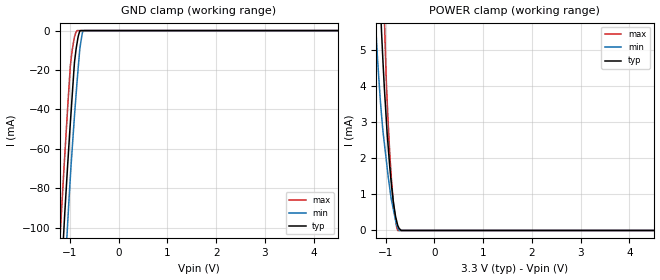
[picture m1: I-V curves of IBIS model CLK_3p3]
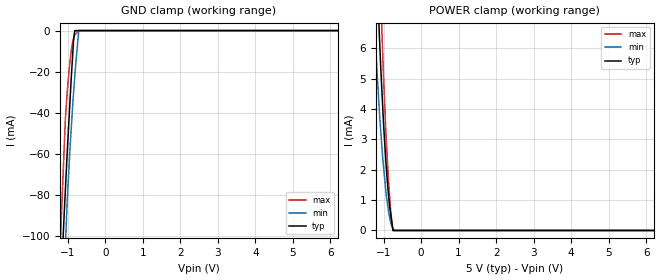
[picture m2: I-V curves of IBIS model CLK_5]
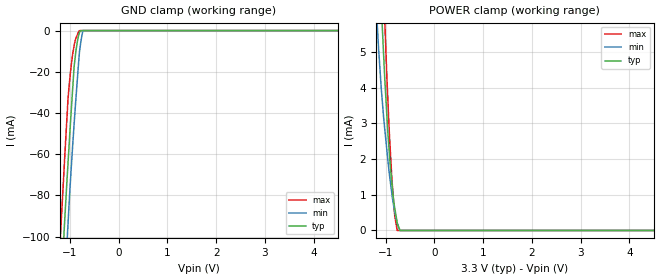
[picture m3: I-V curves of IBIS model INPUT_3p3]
|Texas Instruments Incorporated
|20 Bit Delta Sigma ADC for Bridge Sensors
| Marketing part#   Digital Voltage Range   Package-type   #pins
| ADS1230IPW   2.7V to 5.3V   TSSOP   16
| ADS1230IPWG4   2.7V to 5.3V   TSSOP   16
| ADS1230IPWR   2.7V to 5.3V   TSSOP   16
| ADS1230IPWRG4   2.7V to 5.3V   TSSOP   16
[IBIS Ver]   3.2
[File name]   ads1230.ibs
[Date]   07/16/2010
[File Rev]   1.2
[Source]
| Texas Instruments Incorporated.
| Analog eLab Design Center, HPA
| 12500 TI Blvd
| Dallas, TX -75243
| e-Mail: elab_scm_ibis@list.ti.com
| Model generated from simulations in TISPICE
[Notes]   Revision_History:
|   Rev 1.0: 05/25/2010
|   - Initial version of the model
|   - Initial Model generated from simulations in TIspiceD
|   - Model names with a trailing _3p3 contains the model for
|   3.3V [3 - 3.3 - 3.6]. Model names with trailing _5 contains
|   the model for 5V [4.75 - 5.0 - 5.25] operation.
|   Rev 1.1: 07/08/2010
|   - Model generated from simulations in TISPICE
|   - Model matched to SPICE simulation
|   - Updated the ibis file with data sheet title and package
|   details
|   - While calculating R_pkg, L_pkg and C_pkg ignored values
|   corresponding to power and ground pins
|   - Added package details beside [Package]
|   - C_comp although listed in numerical order of value are
|   obtained from varying PVT conditions. For PVT conditions
|   for each specific value refer the buffer description under
|   respective [Model]. IBIS model user is responsible for using
|   appropriate C_comp to simulate for Signal Integrity.
|   - Removed C_comp (ON state) and C_comp (OFF state) lines
|   Rev 1.2: 07/16/2010
|   - Updated the ibis file with Vinl and Vinh values calculated
|   using VDD typ values and also added model spec
|   - Added C_comp (ON state) and C_comp (OFF state) for OUTPUT_3p3
|   and OUTPUT_5 models
|   - Removed the out of range(-VDD to 2*VDD) voltages for clamp
|   and IV curves
[Disclaimer]
| This model is designed as an aid for customers of Texas Instruments.
| TI and its licensors and suppliers make no warranties, either expressed
| or implied, with respect to this  model, including the warranties of
| merchantability or fitness for a particular purpose. The model is
| provided solely on an "as is" basis. The entire risk as to its quality
| and performance is with the customer.
[Copyright]
| (C) Copyright 2010 Texas Instruments Incorporated. All rights reserved.
|   ADS1230
[Component]   ADS1230
[Manufacturer]  TI
[Package]  | 16 TSSOP - PW package
| variable   typ   min   max
R_pkg   0.07499   0.06418   0.0858
L_pkg   2.774805nH   2.2398nH   3.30981nH
C_pkg   0.48029pF   0.44652pF   0.51406pF
|-------------------------PIN------------------------------------------------
[Pin]  signal_name model_name   R_pin   L_pin   C_pin
1   DVDD   POWER   0.07591   3.10169nH   0.50422pF
2   DGND   GND   0.08317   2.62701nH   0.45709pF
3   CLKIN   CLK   0.06418   2.24125nH   0.45226pF
4   GAIN   INPUT   0.06418   2.23980nH   0.45110pF
5   CAP   TERM   0.06537   2.26241nH   0.45379pF
6   CAP   TERM   0.06501   2.25855nH   0.45528pF
7   AINP   TERM   0.07204   2.40738nH   0.44652pF
8   AINN   TERM   0.06723   2.93633nH   0.49461pF
9   REFN   TERM   0.08580   3.30981nH   0.51406pF
10   REFP   TERM   0.08477   2.66411nH   0.46463pF
11   AGND   GND   0.03843   2.07247nH   0.50509pF
12   AVDD   POWER   0.06944   2.34570nH   0.45854pF
13   SPEED   INPUT   0.06997   2.35644nH   0.46010pF
14   _PDWN   INPUT   0.06418   2.24133nH   0.45470pF
15   SCLK   INPUT   0.08390   2.64189nH   0.45754pF
16   _DRDY/DOUT  OUTPUT   0.07852   3.15400nH   0.50637pF
|   Model Selectors
[Model Selector]  CLK
CLK_3p3   3V digital input
CLK_5   5V digital input
|NOTES   Model CLK split into two Models CLK_3p3 and CLK_5
|   to accomodate vast voltage range of 2.7V - 5.3V
|   CLK_3p3 operates in voltage range of 3.0 - 3.3 - 3.6
|   CLK_5 operates in voltage range of 4.75 - 5.0 - 5.25
|   The max pin frequency for Model CLK is 6MHz
|   This is referenced with CLKIN pin in datasheet
[Model Selector]  INPUT
INPUT_3p3  3V digital input
INPUT_5   5V digital input
|NOTES   Model INPUT split into two Models INPUT_3p3 and INPUT_5
|   to accomodate vast voltage range of 2.7V - 5.3V
|   INPUT_3p3 operates in voltage range of 3.0 - 3.3 - 3.6
|   INPUT_5 operates in voltage range of 4.75 - 5.0 - 5.25
|   The max pin frequency for Model INPUT is 5MHz
|   This is referenced with SCLK pin in datasheet
[Model Selector]  OUTPUT
OUTPUT_3p3   3V digital output
OUTPUT_5   5V digital output
|NOTES   Model OUTPUT split into two Models OUTPUT_3p3 and OUTPUT_5
|   to accomodate vast voltage range of 2.7V - 5.3V
|   OUTPUT_3p3 operates in voltage range of 3.0 - 3.3 - 3.6
|   OUTPUT_5 operates in voltage range of 4.75 - 5.0 - 5.25
|   The max pin frequency for Model OUTPUT is 2.5MHz
|   This is referenced with timing diagrams of _DRDY/DOUT pin
|   in datasheet
|   TERM Model
[Model] TERM
Model_type Terminator
C_comp   0   0   0
| variable   typ   min   max
[Voltage Range]   3.3V   2.7V   5.3V
[POWER Clamp Reference]  3.3V   2.7V   5.3V
[GND Clamp Reference]   0.0V   0.0V   0.0V
|Operating Temperature
[Temperature Range]   25   85   -40
| Models and submodels in the file (7): TERM (Terminator), CLK_3p3 (Input), CLK_5 (Input), INPUT_3p3 (Input), INPUT_5 (Input), OUTPUT_3p3 (Output), OUTPUT_5 (Output)
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|   CLK INPUT 3V Model
[Model]   CLK_3p3
Model_type Input
| Signals  CLK
Vinl = 0.66
Vinh = 2.31
|   typ   min   max
|   (nom PVT)   (Fast PVT)   (slow PVT)
|Average
C_comp   1.099e-12   1.076e-12   1.134e-12
| Where   nom PVT is  Nominal Process, 3.3V, 25C
|   Fast PVT is Strong Process, 3.6V, -40C
|   Slow PVT is Weak Process, 3.0V, 85C
[model spec]
Vinl   0.66   0.6   0.72
Vinh   2.31   2.1   2.52
[Voltage Range]   3.3   3   3.6
|Ambient Temperature   25   85   -40
|Junction Temperature
[Temperature Range]   25   85   -40
[Power Clamp Reference]   3.3   3   3.6
[GND Clamp Reference]   0   0   0
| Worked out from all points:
|   GND clamp passes 1 mA (typ) near -0.81 V on its own axis
|   POWER clamp passes 1 mA (typ) near -0.86 V on its own axis
[GND Clamp]
|   Voltage   I(typ)   I(min)   I(max)
-3.3V     -1.171A    -1.197A    -1.147A
-1.191V   -132.1mA   -162.7mA   -99.85mA
-1.118V   -98.63mA   -129.9mA   -68.62mA
-1.056V   -72.27mA   -102.2mA   -43.23mA
-992.4mV  -47.42mA   -74.93mA   -18.44mA
-978mV    -42.17mA   -69.13mA   -15.05mA
-907.5mV  -16.46mA   -43.73mA   -3.436mA
-848.4mV  -5.674mA   -24.53mA   0A
-795mV    -229.2uA   -8.925mA   0A
-744mV    0A         -1.21mA    0A
-709.5mV  0A         0A         0A
6.6V      0A         0A         0A
[POWER Clamp]
|   Voltage   I(typ)   I(min)   I(max)
-3.3V     108.4mA    89.11mA    133.8mA
-1.201V   9.77mA     5.568mA    14.15mA
-1.164V   8.324mA    4.662mA    12.26mA
-1.089V   5.584mA    3.231mA    8.654mA
-1.03V    3.971mA    2.425mA    5.949mA
-956.4mV  2.424mA    1.567mA    3.148mA
-888mV    1.329mA    875.9uA    1.498mA
-837.6mV  725.4uA    540.1uA    687.9uA
-780mV    281.4uA    156.3uA    122.9uA
-755.7mV  144.4uA    72.09uA    0A
-682.8mV  0A         0A         0A
6.6V      0A         0A         0A
|   CLK INPUT 5V Model
[Model] CLK_5
Model_type Input
| Signals   CLK
Vinl = 1
Vinh = 3.5
|   typ   min   max
|   (nom PVT)   (Fast PVT)   (slow PVT)
|Average
C_comp   1.002e-12   9.906e-13   1.026e-12
| Where   nom PVT is  Nominal Process, 5.0V, 25C
|   Fast PVT is Strong Process, 5.25V, -40C
|   Slow PVT is Weak Process, 4.75V, 85C
[model spec]
Vinl   1   0.95   1.05
Vinh   3.5   3.325   3.675
[Voltage Range]   5   4.75   5.25
|Ambient Temperature   25   85   -40
|Junction Temperature
[Temperature Range]   25   85   -40
[Power Clamp Reference]   5   4.75   5.25
[GND Clamp Reference]   0   0   0
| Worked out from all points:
|   GND clamp passes 1 mA (typ) near -0.82 V on its own axis
|   POWER clamp passes 1 mA (typ) near -0.86 V on its own axis
[GND Clamp]
|   Voltage   I(typ)   I(min)   I(max)
-5V       -2.025A    -2.047A    -2.006A
-1.183V   -128.3mA   -159.9mA   -97.69mA
-1.145V   -110.4mA   -142.7mA   -80.53mA
-1.1V     -92.25mA   -122.5mA   -60.34mA
-1.057V   -76.17mA   -103.3mA   -42.31mA
-1.026V   -64.45mA   -89.13mA   -33.61mA
-947mV    -37.4mA    -60.77mA   -16.42mA
-894.5mV  -20.28mA   -44.76mA   -8.557mA
-845mV    -5.353mA   -30.81mA   -3.951mA
-810.5mV  0A         -22.1mA    -1.985mA
-701.3mV  0A         -664.7nA   0A
10V       0A         0A         0A
[POWER Clamp]
|   Voltage   I(typ)   I(min)   I(max)
-5V       191mA      160.6mA    232.8mA
-1.245V   11.62mA    7mA        16.59mA
-1.13V    7.008mA    4.333mA    10.7mA
-1.105V   6.248mA    3.805mA    9.425mA
-1.052V   4.809mA    2.897mA    6.857mA
-1.02V    4.004mA    2.346mA    5.737mA
-995mV    3.409mA    2.032mA    4.917mA
-936.5mV  2.248mA    1.281mA    3.217mA
-878.8mV  1.327mA    735.6uA    1.863mA
-810.5mV  546.5uA    267.7uA    662.3uA
-750mV    0A         90.21uA    917.7nA
10V       0A         0A         0A
|   Input INPUT 3V Model
[Model] INPUT_3p3
Model_type Input
| Signals   GAIN(4), SPEED(13), _PWDN(14), SCLK(15)
Vinl = 0.66
Vinh = 2.31
|   typ   min   max
|   (nom PVT)   (Fast PVT)   (slow PVT)
|Average
C_comp   9.839e-13   9.531e-13   9.951e-13
| Where   nom PVT is  Nominal Process, 3.3V, 25C
|   Fast PVT is Strong Process, 3.6V, -40C
|   Slow PVT is Weak Process, 3.0V, 85C
[model spec]
Vinl   0.66   0.6   0.72
Vinh   2.31   2.1   2.52
[Voltage Range]   3.3   3   3.6
|Ambient Temperature   25   85   -40
|Junction Temperature
[Temperature Range]   25   85   -40
[Power Clamp Reference]   3.3   3   3.6
[GND Clamp Reference]   0   0   0
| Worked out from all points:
|   GND clamp passes 1 mA (typ) near -0.80 V on its own axis
|   POWER clamp passes 1 mA (typ) near -0.85 V on its own axis
[GND Clamp]
|   Voltage   I(typ)   I(min)   I(max)
-3.3V     -1.162A    -1.19A     -1.135A
-1.191V   -130.5mA   -161.6mA   -98.4mA
-1.187V   -128.5mA   -159.7mA   -96.51mA
-1.115V   -95.82mA   -127.7mA   -65.41mA
-1.056V   -71.21mA   -101.4mA   -40.4mA
-1.039V   -64.61mA   -94.11mA   -33.37mA
-974.4mV  -39.65mA   -67.39mA   -17.17mA
-910.8mV  -16.92mA   -44.44mA   -6.948mA
-874.5mV  -9.538mA   -32.39mA   -3.596mA
-804mV    -951.7uA   -10.49mA   0A
-729.6mV  0A         0A         0A
6.6V      0A         0A         0A
[POWER Clamp]
|   Voltage   I(typ)   I(min)   I(max)
-3.3V     115.2mA    94.41mA    142.9mA
-1.2V     10.66mA    6.386mA    15.13mA
-1.152V   8.635mA    5.203mA    12.51mA
-1.073V   5.727mA    3.643mA    8.36mA
-1.02V    4.222mA    2.825mA    5.846mA
-957mV    2.742mA    1.97mA     3.658mA
-924mV    2.098mA    1.556mA    2.651mA
-873.6mV  1.314mA    1.015mA    1.423mA
-816mV    631.6uA    508.2uA    417.1uA
-765.6mV  216.4uA    202.3uA    0A
-708mV    19.17nA    0A         0A
6.6V      0A         0A         0A
